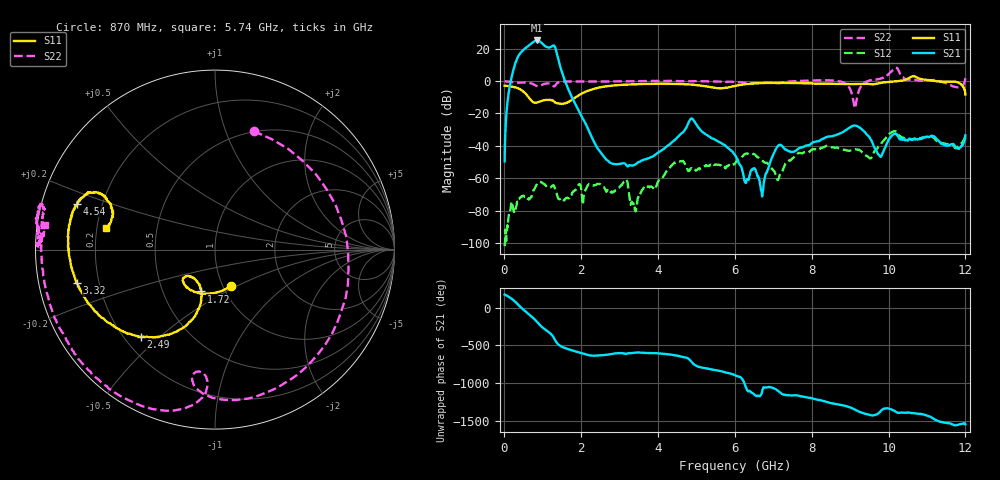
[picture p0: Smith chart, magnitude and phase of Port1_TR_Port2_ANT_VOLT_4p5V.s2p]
! Created Mon Aug 25 11:01:56 2025
# hz S ma R 50
! 2 Port Network Data from SP1.SP block
! freq  magS11  angS11  magS21  angS21  magS12  angS12  magS22  angS22
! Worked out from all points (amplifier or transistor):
!   1200 points, 10 MHz to 12 GHz, reference 50 ohm
!   highest |S21| = 25.0 dB at 860 MHz (marker M1)
!   |S21| within 3 dB of that: 644.2 MHz to 1.039 GHz (394.8 MHz wide, 46.9 % of centre)
!   unconditionally stable (mu >= 1): start of sweep to 3.538 GHz; 4.513 GHz to 7.641 GHz; 8.673 GHz to 9.462 GHz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
!   at 2.01 GHz: K = 752.80, MAG = -8.7 dB, |S12| = -67.8 dB
!   at 6.01 GHz: K = 2063.37, MAG = -33.7 dB, |S12| = -50.7 dB
!   at 12 GHz: K = -840.73, MSG = -0.6 dB, |S12| = -32.4 dB
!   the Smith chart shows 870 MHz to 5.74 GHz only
!   S11 on the Smith chart (normalised r, x): 870 MHz: 1.09, -0.47; 1.72 GHz: 0.77, -0.38; 2.49 GHz: 0.26, -0.44; 3.32 GHz: 0.12, -0.12; 4.54 GHz: 0.11, +0.16; 5.74 GHz: 0.24, +0.09
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1e7  0.717 178.6  0.003323 172.1  8.115e-06 -90.7  0.9836 176.3
3.4e8  0.609 128.5  5.032 49.5  0.0001922 132.3  0.8923 9.8
5.1e8  0.4606 89.1  9.374 -31.6  0.0002791 89.9  0.9034 -94.4
7.1e8  0.2469 11.2  14.53 -116.3  0.0002747 103.3  0.8435 -178.4
8e8  0.2138 -34.5  17.11 -159.9  0.0005126 95.6  0.7523 128.9
8.6e8  0.2194 -62.0  17.84 167.3  0.000704 77.4  0.6967 80.6
8.7e8  0.2227 -66.1  17.76 161.7  0.0007287 73.7  0.6944 71.8
1e9  0.2506 -101.5  13.87 95.7  0.0007054 25.8  0.7817 -25.4
1.22e9  0.2592 -130.9  11.35 9.5  0.0005477 -27.2  0.8047 -94.8
1.32e9  0.2188 -137.6  11.21 -66.8  0.0004873 -104.3  0.7081 -94.1
1.41e9  0.2053 -132.8  4.544 -128.0  0.000239 -158.2  0.9127 -102.6
1.72e9  0.2456 -108.4  0.4049 161.7  0.0002564 145.4  0.9743 -133.6
2.01e9  0.4075 -107.8  0.08254 118.8  0.0004086 61.4  0.9691 -151.7
2.49e9  0.6394 -130.4  0.006686 89.3  0.0006621 58.8  0.9673 -174.9
3.32e9  0.7928 -166.4  0.002507 119.5  0.0001906 -0.9  0.9856 166.2
4.01e9  0.8226 172.8  0.006327 115.6  0.0008401 76.2  1.009 167.3
4.54e9  0.8094 161.5  0.02021 81.4  0.003314 7.2  0.9902 172.6
5.74e9  0.617 168.8  0.01058 -132.5  0.002207 -25.4  0.9571 171.8
6.01e9  0.7059 175.9  0.005163 -174.0  0.002933 -3.8  0.9357 159.2
8.01e9  0.8416 159.4  0.01233 -116.6  0.007688 -93.3  1.041 56.2
1.001e10  0.9377 127.7  0.01603 105.5  0.02284 133.2  1.669 136.9
1.2e10  0.3862 75.2  0.02113 -101.0  0.02404 -84.9  1.415 64.1
